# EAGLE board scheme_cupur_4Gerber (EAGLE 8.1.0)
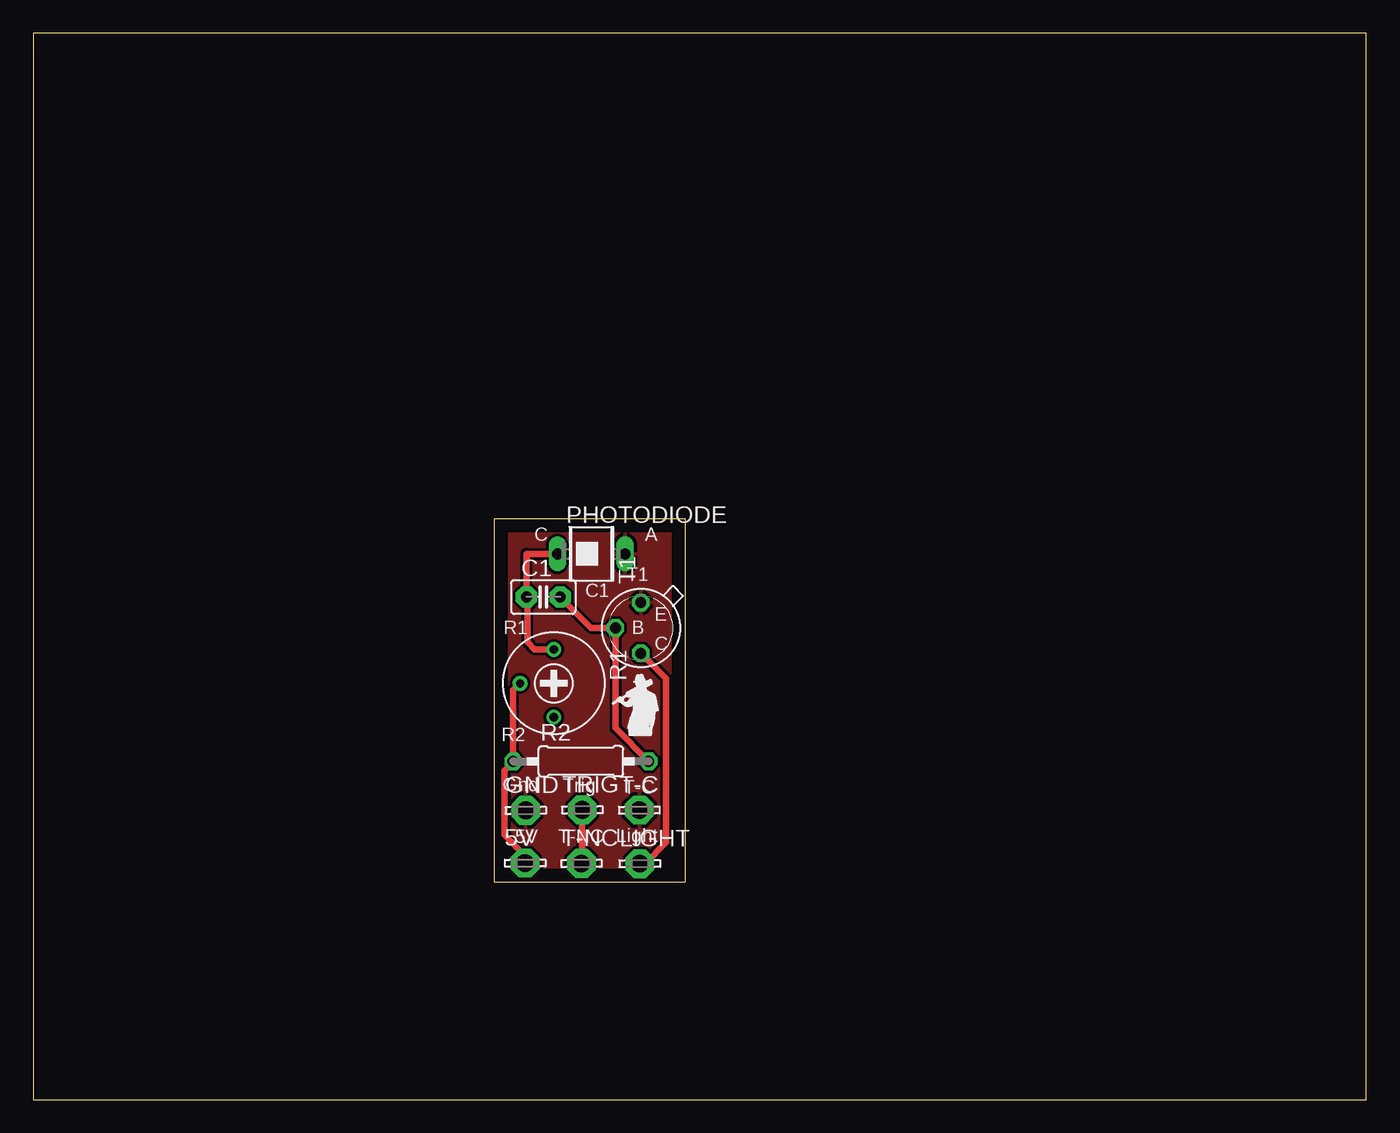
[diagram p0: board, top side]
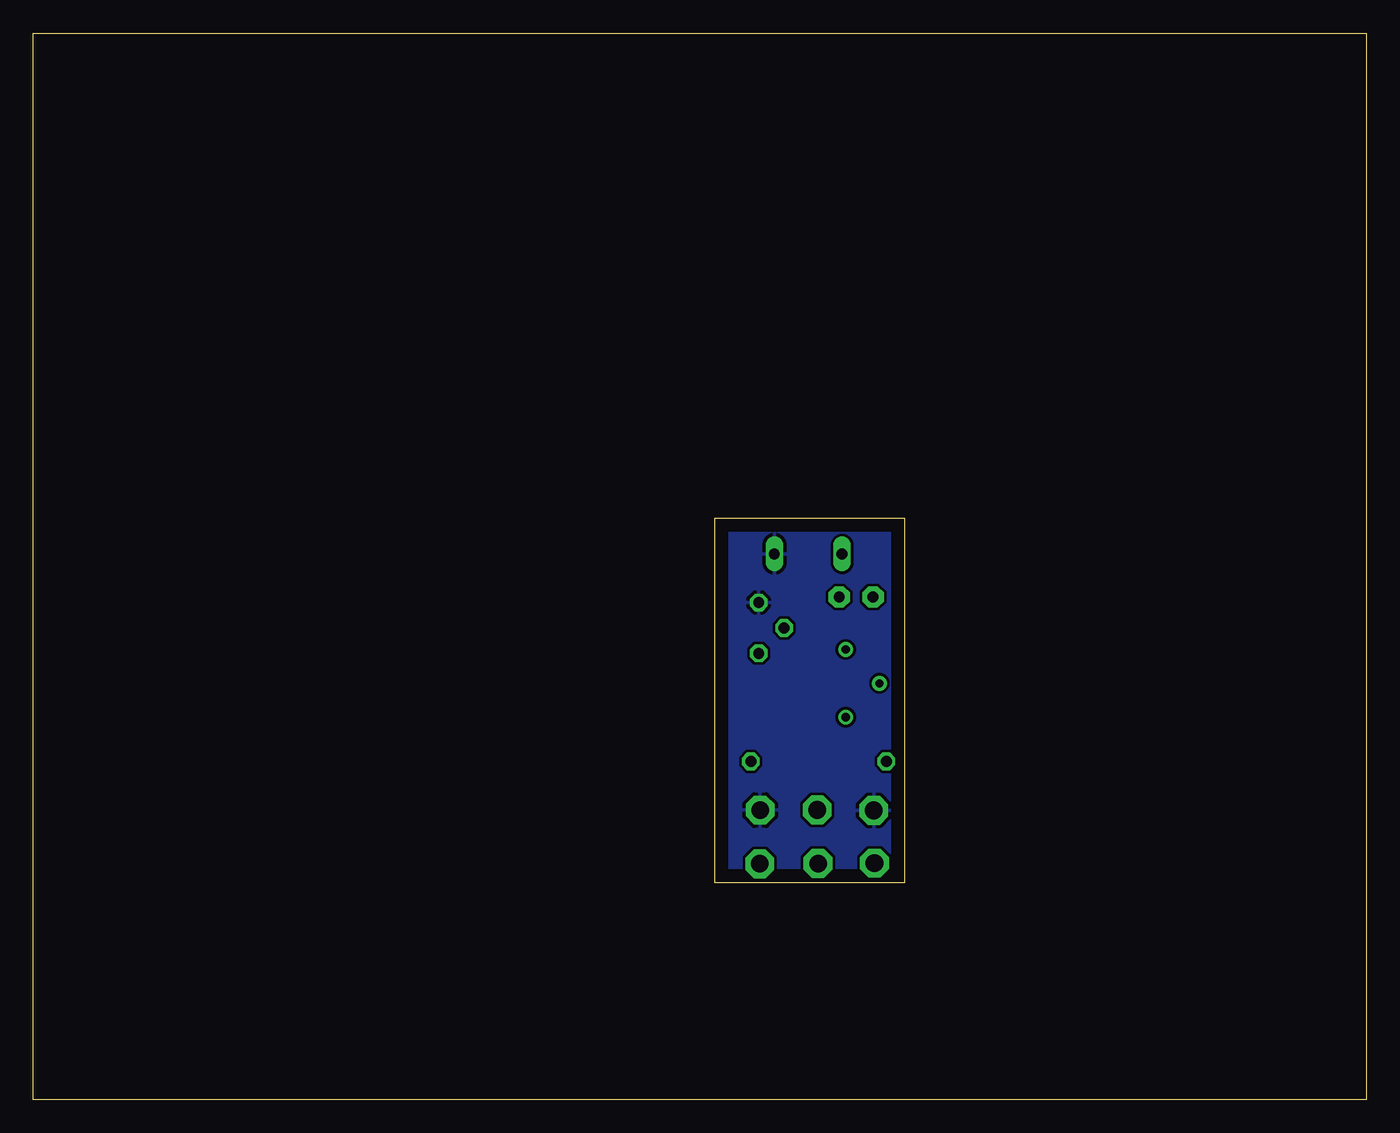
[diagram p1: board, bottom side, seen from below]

Size 100 x 80 mm. Coordinates in mm from the lower left corner, seen from the top.
Outline: 0,0 100,0 100,80 0,80 0,0
Outline: 34.6,43.6 48.9,43.6 48.9,16.3 34.6,16.3 34.6,43.6
Copper layers (1*16): Top 0.035mm / dielectric 1.5mm / Bottom 0.035mm
Design rules "default": minimum track width 10mil, minimum drill 24mil, track to track 8mil, track to pad 8mil, pad to pad 8mil, via to via 8mil, smd to smd 8mil, copper to edge 40mil, drill to drill 8mil, minimum pad ring 10mil, minimum via ring 8mil, stop-mask expansion 4mil, vias tented up to drill 0mil, thermal gap 10mil

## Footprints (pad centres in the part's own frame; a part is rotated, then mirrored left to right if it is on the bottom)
LSP13 = drill 1.321 pad 2.159 octagon: MP 0,0
C2.5-2 = drill 0.813 pad 1.6 octagon: 1 -1.27,0; 2 1.27,0
BP104 = drill 0.813 long: A 0,2.54; K 0,-2.54
RTRIM3339P = drill 0.61: 1 -2.54,0; 2 0,-2.54; 3 2.54,0
0207/10 = drill 0.813 octagon: 1 -5.08,0; 2 5.08,0
TO18- = drill 0.813 octagon: 1 1.905,0; 2 0,1.905; 3 -1.905,0

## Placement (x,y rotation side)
5V  LSP13  [LSP13]  36.89,17.74 0 top
C1  0.1uF  [C2.5-2]  38.27,37.71 0 top
GND  LSP13  [LSP13]  36.94,21.7 0 top
LIGHT  LSP13  [LSP13]  45.5,17.69 0 top
PHOTODIODE  5800B  [BP104]  41.87,40.94 270 top
R1  0-10 kOhm  [RTRIM3339P]  39.05,31.23 270 top
R2  1 kOhm  [0207/10]  41.08,25.37 0 top
T1  2N3904  [TO18-]  45.58,35.38 90 top
T-C  LSP13  [LSP13]  45.47,21.72 0 top
T-NC  LSP13  [LSP13]  41.13,17.71 0 top
TRIG  LSP13  [LSP13]  41.19,21.73 0 top

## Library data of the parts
5V GND LIGHT T-C T-NC TRIG = solpad
C1 = capacitor-wima
PHOTODIODE = opto-trans-siemens; MF: VISHAY/TELEFUNKEN; MPN: BP104; OC_FARNELL: 1779636; OC_NEWARK: 14M4504
R1 = rcl
R2 = eagle-ltspice; SPICEMODEL: NONE; SPICEPREFIX: R
T1 = transistor

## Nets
GND: GND.MP PHOTODIODE.A T1.1 T-C.MP
N$1: LIGHT.MP T1.3
N$2: C1.2 R2.2 T1.2
N$4: 5V.MP R1.2 R2.1
N$5: C1.1 PHOTODIODE.K R1.1
N$6: T-NC.MP TRIG.MP

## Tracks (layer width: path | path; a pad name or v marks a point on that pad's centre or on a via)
GND
  pour Top (isolate 0.15): 34.6,43.6 48.9,43.6 48.9,43.4 48.9,16.3 34.6,16.3 34.6,16.7
  pour Bottom (isolate 0.15): 34.6,43.6 48.9,43.6 48.9,43.3 48.9,16.3 34.6,16.3 34.6,16.4
N$1
  Top 0.406: 47.48,19.5 47.48,19.29 arc-45 47.48,19.28
  Top 0.5: T1.3 47.48,31.58 47.48,19.5 | LIGHT.MP 45.89,17.69 47.48,19.28
N$2
  Top 0.5: C1.2 41.86,35.38 T1.2 43.67,27.87 R2.2
N$4
  Top 0.5: R2.1 36.01,25.32 35.87,25.18 | 5V.MP 36.89,18.29 35.34,19.84 35.34,24.71 R2.1 | R2.1 36.01,30.72 R1.2
N$5
  Top 0.5: C1.1 37.12,37.46 37.07,37.41 37.07,34.31 37.62,33.77 R1.1 | 36.69,38.01 C1.1 | C1.1 36.99,40.94 PHOTODIODE.K
N$6
  Top 0.5: T-NC.MP 41.19,17.78 TRIG.MP

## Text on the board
tPlace: C | A | T1 | C1 | E | R1 | B | C | R2 | Gnd | Trig | T-C | 5V | T-NC | Light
